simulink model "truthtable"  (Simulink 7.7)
settings: Solver=FixedStepDiscrete  StartTime=0.0  StopTime=7  FixedStep=0.1  RelTol=1e-3
libraries: simulink x1

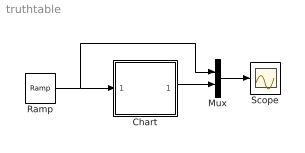
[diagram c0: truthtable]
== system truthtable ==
  Chart : Stateflow chart  TreatAsAtomicUnit=on
  Mux : Mux  Inputs=2
  Ramp : simulink/Sources/Ramp  SystemSampleTime=-1  slope=1  start=0  X0=0
  Scope : Scope
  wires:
  Ramp/1 -> Chart/1(in), Mux/1
  Chart/1(out) -> Mux/2
  Mux/1 -> Scope/1

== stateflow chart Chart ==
  state y = f(x) [function]
    (default) -> (junction 5)
    (junction 5) -> (junction 6) : { /* erste Stufe */ LOWER_SAT = (x<1); }
    (junction 6) -> (junction 7) : { /* zweite Stufe */ aVarTruthTableCondition_2 = (x<2); }
    (junction 7) -> (junction 8) : { /* dritte Stufe */ aVarTruthTableCondition_3 = (x<3); }
    (junction 8) -> (junction 9) : { /* vierte Stufe */ aVarTruthTableCondition_4 = (x<4); }
    (junction 9) -> (junction 10) : { /* fünfte Stufe */ UPPER_SAT = (x<5); }
    (junction 10) -> (junction 11) : [LOWER_SAT && aVarTruthTableCondition_2 && aVarTruthTableCondition_3 && aVarTruthTableCondition_4 && UPPER_SAT]
    (junction 11) -> (junction 12) : { /* 'zero':setze y auf 0 */ y=0; }
    (junction 10) -> (junction 13)
    (junction 13) -> (junction 14) : [!LOWER_SAT && aVarTruthTableCondition_2 && aVarTruthTableCondition_3 && aVarTruthTableCondition_4 && UPPER_SAT]
    (junction 14) -> (junction 15) : { /* setze y auf 1 */ y=1; }
    (junction 13) -> (junction 16)
    (junction 16) -> (junction 17) : [!LOWER_SAT && !aVarTruthTableCondition_2 && aVarTruthTableCondition_3 && aVarTruthTableCondition_4 && UPPER_SAT]
    (junction 17) -> (junction 18) : { /* setze y auf 2 */ y=2; }
    (junction 16) -> (junction 19)
    (junction 19) -> (junction 20) : [!LOWER_SAT && !aVarTruthTableCondition_2 && !aVarTruthTableCondition_3 && aVarTruthTableCondition_4 && UPPER_SAT]
    (junction 20) -> (junction 21) : { /* setze y auf 3 */ y=3; }
    (junction 19) -> (junction 22)
    (junction 22) -> (junction 23) : [!LOWER_SAT && !aVarTruthTableCondition_2 && !aVarTruthTableCondition_3 && !aVarTruthTableCondition_4 && UPPER_SAT]
    (junction 23) -> (junction 24) : { /* setze y auf 4 */ y=4; }
    (junction 22) -> (junction 25)
    (junction 25) -> (junction 26) : /* Default */
    (junction 26) -> (junction 27) : { /* setze y auf 5 */ y=5; }
  (default) -> (junction 4) : {out=f(in);}
